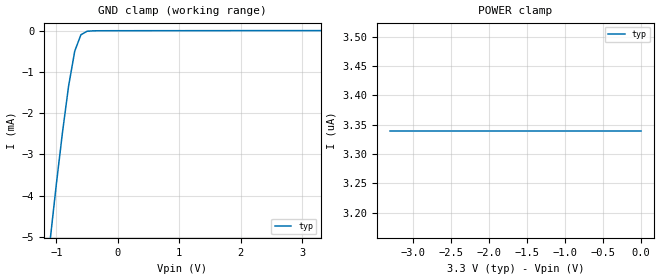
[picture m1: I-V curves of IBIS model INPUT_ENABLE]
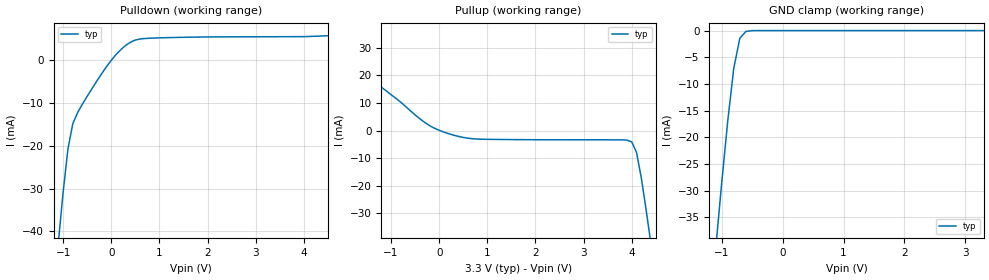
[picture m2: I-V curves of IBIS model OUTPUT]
|   Texas Instruments Incorporated
|   Data Transmissions Products
|   IBIS Model for SN65LVDS389
|   38DBT TSSOP Package
[IBIS Ver]   2.1
[Comment char]   |_char
[File name]   lvds389.ibs
[File Rev]   1.0
[Date]   12Jan00
[Source]   File originated at Texas Instruments Incorporated.
   Data Transmission Products Group.
[Notes]
[Disclaimer]
(C) Copyright Texas Instruments Incorporated 2000
   All rights reserved
  Texas Instruments Incorporated hereby grants the user of this IBIS
model a non-exclusive, nontransferable license to use this IBIS model
under the following terms.  Before using this IBIS model, the user
should read this license.  If the user does not accept these terms,
the IBIS model should be returned to Texas Instruments within 30 days.
  The user is granted this license only to use the IBIS model and
is not granted rights to sell, load, rent, lease or license the IBIS
model in whole or in part, or in modified form to anyone other than
user.  User may modify the IBIS model to suit its specific applications
but rights to derivative works and such modifications shall belong to
Texas Instruments.
  This IBIS model is provided on an "AS IS" basis and Texas Instruments
makes absolutely no warranty with respect to the information contained
herein.  TEXAS INSTRUMENTS DISCLAIMS AND CUSTOMER WAIVES ALL WARRANTIES,
EXPRESS OR IMPLIED, INCLUDING WARRANTIES OF MERCHANTABILITY OR FITNESS
FOR A PARTICULAR PURPOSE. The entire risk as to quality and performance
is with the Customer. ACCORDINGLY, IN NO EVENT SHALL THE COMPANY BE LIABLE
FOR ANY DAMAGES, WHETHER IN CONTRACT OR TORT,INCLUDING ANY LOST PROFITS
OR OTHER INCIDENTAL, CONSEQUENTIAL, EXEMPLARY, OR PUNITIVE DAMAGES ARISING
OUT OF THE USE OR APPLICATION OF THE IBIS model provided in this package.
Further, Texas Instruments reserves the right to discontinue or make changes
without notice to any product herein to improve reliability, function, or
design. Texas Instruments does not convey any license under patent rights
or any other intellectual property rights, including those of third parties.
Contact Texas Instruments at ATTN:DATA TRANSMISSIONS
Thomas Fisher 12500 TI Boulevard, M/S 8710  Dallas, Texas 75243
[Copyright]   Copyright 2000, Texas Instruments, All Rights Reserved
[Component]   LVDS389DGG
[Manufacturer]  Texas Instruments Incorporated
[Package]
|   typ   min   max
R_pkg   0.040   0.035   0.047
L_pkg   2.433nH   1.956nH   3.508nH
C_pkg   0.451pF   0.362pF   0.635pF
[Pin]   signal_name   model_name   R_pin   L_pin   C_pin
1   GND   GND   0.047   3.508n   0.598p
2   VCC   POWER   0.047   3.231n   0.634p
3   GND   GND   0.046   2.932n   0.570p
4   ENA   INPUT_ENABLE   0.043   2.459n   0.459p
5   A1A   INPUT_ENABLE   0.035   2.103n   0.387p
6   A2A   INPUT_ENABLE   0.036   2.005n   0.369p
7   A3A   INPUT_ENABLE   0.035   1.956n   0.365p
8   A4A   INPUT_ENABLE   0.036   1.965n   0.364p
9   GND   GND   0.036   1.965n   0.363p
10   VCC   POWER   0.036   1.974n   0.362p
11   GND   GND   0.036   1.965n   0.362p
12   B1A   INPUT_ENABLE   0.036   1.965n   0.364p
13   B2A   INPUT_ENABLE   0.036   1.956n   0.365p
14   B3A   INPUT_ENABLE   0.036   2.005n   0.369p
15   B4A   INPUT_ENABLE   0.035   2.102n   0.387p
16   ENB   INPUT_ENABLE   0.043   2.459n   0.459p
17   GND   GND   0.046   2.932n   0.570p
18   VCC   POWER   0.047   3.231n   0.634p
19   GND   GND   0.047   3.508n   0.598p
20   B4Z   OUTPUT   0.047   3.508n   0.598p
21   B4Y   OUTPUT   0.047   3.231n   0.634p
22   B3Z   OUTPUT   0.046   2.932n   0.570p
23   B3Y   OUTPUT   0.043   2.459n   0.458p
24   B2Z   OUTPUT   0.035   2.103n   0.387p
25   B2Y   OUTPUT   0.036   2.005n   0.369p
26   B1Z   OUTPUT   0.035   1.956n   0.365p
27   B1Y   OUTPUT   0.036   1.965n   0.364p
28   NC   NC
29   NC   NC
30   NC   NC
31   A4Z   OUTPUT   0.036   1.965n   0.364p
32   A4Y   OUTPUT   0.036   1.956n   0.365p
33   A3Z   OUTPUT   0.036   2.004n   0.369p
34   A3Y   OUTPUT   0.035   2.102n   0.387p
35   A2Z   OUTPUT   0.043   2.459n   0.458p
36   A2Y   OUTPUT   0.046   2.932n   0.570p
37   A1Z   OUTPUT   0.047   3.231n   0.635p
38   A1Y   OUTPUT   0.047   3.508n   0.598p
[Diff_pin]   inv_pin   vdiff   tdelay_typ   tdelay_min   tdelay_max
| The 'xY' pin is Diff_pin and the 'xZ' pin is the inv_pin
21   20   NA   0 0 0
23   22   NA   0 0 0
25   24   NA   0 0 0
27   26   NA   0 0 0
32   31   NA   0 0 0
34   33   NA   0 0 0
36   35   NA   0 0 0
38   37   NA   0 0 0
| Models and submodels in the file (2): INPUT_ENABLE (Input), OUTPUT (3-state)
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|   Driver Input / Enable Model
[Model]   INPUT_ENABLE
Model_type   Input
|Signals   A1A,A2A,A3A,A4A,B1A,B2A,B3A,B4A
|   ENA,ENB,ENC,END
Vinh = 2.0
Vinl = 0.8
|   typ   min   max
C_comp   1.0pF   NA   NA
|   typ   min   max
[Temperature Range]   25.0   NA   NA
[Voltage range]   3.3V   3.0V   3.6V
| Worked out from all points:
|   GND clamp passes 1 mA (typ) near -0.76 V on its own axis
[GND_clamp]
|   Voltage   I(typ)   I(min)   I(max)
-3.3V     -43.1mA    NA         NA
-1.1V     -5.08mA    NA         NA
-1V       -3.73mA    NA         NA
-900mV    -2.47mA    NA         NA
-800mV    -1.34mA    NA         NA
-700mV    -493uA     NA         NA
-600mV    -98.5uA    NA         NA
-500mV    -13.3uA    NA         NA
3.3V      3.34uA     NA         NA
[Power_clamp]
| Note that the[POWER_clamp]voltage table is referenced to Vcc
| and is calculated using Vtable=Vcc - Vmeasured.
|   Voltage   I(typ)   I(min)   I(max)
-3.3V     3.34uA     NA         NA
-2.7V     3.34uA     NA         NA
-2V       3.34uA     NA         NA
-800mV    3.34uA     NA         NA
0V        3.34uA     NA         NA
|   Driver Output  MODEL
[Model]   OUTPUT
Model_type   3-state
| Signals   A1Y,A1Z,A2Y,A2Z,A3Y,A3Z,A4Y,A4Z,B1Y,B1Z,B2Y,B2Z,B3Y,B3Z,B4Y,B4Z
Vmeas = 1.2V   |Reference voltage for timing measurements
Cref = 5pF   |Timing specification test load capacitance value
Rref = 50   |Note: 50 Ohm load; single ended configuration
Vref = 1.18V   |Timing specification test load voltage
| variable   typ   min   max
C_comp   1.0pF   NA   NA
|   typ   min   max
[Temperature Range]   25.0   NA   NA
[Voltage range]   3.3V   3.0V   3.6V
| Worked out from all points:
|   slope of the pulldown table from 0 to 0.495 V, typ, clamps not added: 105 ohm
|   slope of the pullup table from 0 to 0.495 V, typ, clamps not added: 192 ohm
|   GND clamp passes 1 mA (typ) near -0.67 V on its own axis
[Pulldown]
|   Voltage   I(typ)   I(min)   I(max)
-3.3V     -348mA     NA         NA
-1.1V     -42.6mA    NA         NA
-1V       -30.8mA    NA         NA
-900mV    -20.7mA    NA         NA
-800mV    -14.9mA    NA         NA
-600mV    -10.3mA    NA         NA
-100mV    -1.58mA    NA         NA
200mV     2.42mA     NA         NA
500mV     4.64mA     NA         NA
1.4V      5.26mA     NA         NA
4.1V      5.46mA     NA         NA
6.6V      7.11mA     NA         NA
[Pullup]
|   Voltage   I(typ)   I(min)   I(max)
| Note that the[Pullup]voltage table is referenced to Vcc
| and is calculated using Vtable=Vcc - Vmeasured.
-3.3V     49.3mA     NA         NA
-2.6V     37.7mA     NA         NA
-1.9V     25.6mA     NA         NA
-400mV    4.24mA     NA         NA
200mV     -1.17mA    NA         NA
800mV     -3.11mA    NA         NA
4V        -4.13mA    NA         NA
4.1V      -8.04mA    NA         NA
4.2V      -17.4mA    NA         NA
4.3V      -29mA      NA         NA
4.4V      -41.4mA    NA         NA
6.6V      -348mA     NA         NA
[GND_clamp]
|   Voltage   I(typ)   I(min)   I(max)
| Outputs in High Impedance (off)
-3.3V     -347mA     NA         NA
-1.1V     -41.4mA    NA         NA
-1V       -28.8mA    NA         NA
-900mV    -17.1mA    NA         NA
-800mV    -7.08mA    NA         NA
-700mV    -1.43mA    NA         NA
-600mV    -153uA     NA         NA
-400mV    -866nA     NA         NA
3.3V      -59.7pA    NA         NA
[POWER_clamp]
|   Voltage   I(typ)   I(min)   I(max)
| Note that the [POWER_clamp] voltage table is referenced to Vcc
| and is calculated using Vtable = Vcc - Vmeasured.
| Outputs in Tri-state.
-3.3V     0A         NA         NA
0V        0A         NA         NA
[Ramp]
|   typ   min   max
dV/dt_r   0.346/600ps   NA   NA
dV/dt_f   0.309/600ps   NA   NA
R_load = 100ohm | Note: The measurement is on a differential configuration
